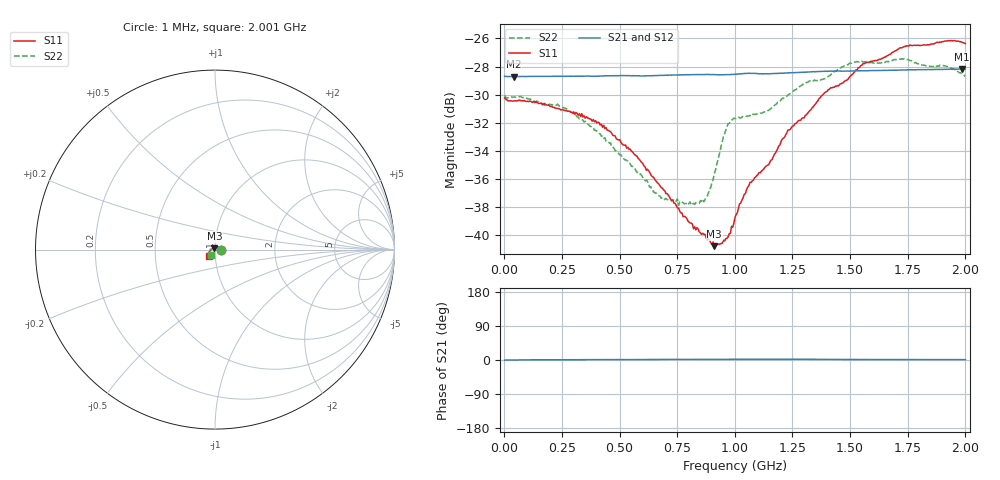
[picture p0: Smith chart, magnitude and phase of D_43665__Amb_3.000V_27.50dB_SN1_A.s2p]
! device id: 43665_
! dir: \\malibu\benchdata\1_engineers\tn_data\43665_75ohm\new\sparar\43665_\amb\3p000v\27p50db
! Serial: 1
! Insertion: A
! Temp: Amb
! VDD: 3.000V
! Attenuation Step: 27.50dB
! IDD: 1.450448e+00mA
! FILE NAME
! DATE 03-27-2009 08:40:08
! CORRECTED  DATA
#  Hz  S  RI  R  75
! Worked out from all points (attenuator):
!   401 points, 1 MHz to 2.001 GHz, reference 75 ohm
!   highest |S21| = -28.17 dB at 1.986 GHz (marker M1); lowest = -28.7 dB at 41 MHz (marker M2)
!   lowest |S11| = -40.8 dB at 911 MHz (marker M3), VSWR 1.02, Z = 74.4 + j1.24 ohm
!   |S11| at or under -10 dB: start of sweep to end of sweep
!   |S22| runs from -37.9 to -27.4 dB; largest |S21 - S12| = 0.00025
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1000000  0.0308 -0.000406  0.0367 -0.000183  0.0368 5.61e-05  0.0315 -9.53e-05
4.1e7  0.03 0.0011  0.0367 5.85e-05  0.0367 7.7e-05  0.031 0.00181
2.41e8  0.0274 0.00626  0.0368 0.000374  0.0368 0.000421  0.0267 0.0107
3.36e8  0.0257 0.00833  0.0368 0.000497  0.0368 0.000541  0.0217 0.0139
4.21e8  0.0224 0.0107  0.0369 0.00067  0.0369 0.0007  0.0167 0.015
5.46e8  0.0168 0.0113  0.0369 0.000689  0.0369 0.000726  0.00895 0.0156
6.71e8  0.00996 0.0114  0.037 0.000954  0.037 0.00101  0.000439 0.0138
8.36e8  0.0013 0.0106  0.0373 0.000994  0.0373 0.00107  -0.0109 0.00709
8.76e8  -0.00145 0.00967  0.0373 0.000987  0.0373 0.00105  -0.0131 0.00387
9.11e8  -0.00381 0.0083  0.0372 0.000939  0.0373 0.00105  -0.0165 0.00148
9.61e8  -0.00655 0.0072  0.0372 0.00111  0.0372 0.0012  -0.0236 0.000464
1.001e9  -0.00948 0.00659  0.0374 0.00123  0.0374 0.00131  -0.0259 0.0019
1.066e9  -0.0147 0.00459  0.0377 0.00108  0.0377 0.00122  -0.0266 -0.00123
1.151e9  -0.018 0.00154  0.0375 0.00116  0.0376 0.00131  -0.0274 -0.00556
1.236e9  -0.0236 -0.0023  0.0378 0.00127  0.0378 0.00139  -0.0298 -0.011
1.336e9  -0.0275 -0.00687  0.0381 0.00124  0.0382 0.00137  -0.0315 -0.0163
1.396e9  -0.0305 -0.0108  0.0383 0.00105  0.0384 0.00125  -0.0302 -0.0199
1.556e9  -0.0358 -0.0194  0.0385 0.000896  0.0386 0.000977  -0.0318 -0.0264
1.671e9  -0.0365 -0.0244  0.0386 0.000795  0.0387 0.000934  -0.0307 -0.0282
1.756e9  -0.0367 -0.0296  0.0387 0.000764  0.0389 0.000771  -0.0286 -0.0308
1.986e9  -0.033 -0.0357  0.039 0.000678  0.0391 0.000643  -0.0233 -0.0293
2.001e9  -0.0323 -0.0355  0.039 0.000671  0.0391 0.000659  -0.0229 -0.0287
